FUNCTION_BLOCK FB_LD_IEDLD1 EXTENDS FB_AcsiCommonLogicalDeviceClass
VAR_INPUT
	LLN0: FB_LN_IED_LD1_LLN0 := (sClass:='LLN0', bLinkResult:=THIS^.AddLogicalNodeToContainer(ipLogicalNode:=LLN0));
	LPHD1: FB_LN_IED_LD1_LPHD1 := (sClass:='LPHD', bLinkResult:=THIS^.AddLogicalNodeToContainer(ipLogicalNode:=LPHD1));
	MMXU1: FB_LN_IED_LD1_MMXU1 := (sClass:='MMXU', bLinkResult:=THIS^.AddLogicalNodeToContainer(ipLogicalNode:=MMXU1));
	XCBR1: FB_LN_IED_LD1_XCBR1 := (sClass:='XCBR', bLinkResult:=THIS^.AddLogicalNodeToContainer(ipLogicalNode:=XCBR1));
END_VAR
VAR
END_VAR

END_FUNCTION_BLOCK
